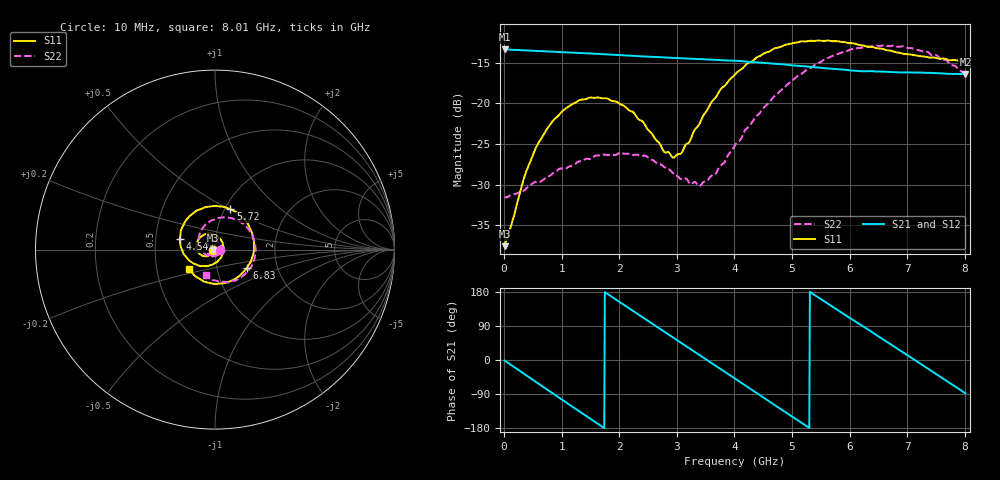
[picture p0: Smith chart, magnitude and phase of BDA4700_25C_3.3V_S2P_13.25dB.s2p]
!Agilent Technologies,E5071B,MY42404982,A.09.10
!Date: Mon Oct 20 18:08:35 2025
!Data & Calibration Information:
!Freq	S11:SOLT2(ON)	S21:SOLT2(ON)	S12:SOLT2(ON)	S22:SOLT2(ON)
# Hz S RI R 50
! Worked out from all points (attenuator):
!   801 points, 10 MHz to 8.01 GHz, reference 50 ohm
!   highest |S21| = -13.35 dB at 10 MHz (marker M1); lowest = -16.4 dB at 8.01 GHz (marker M2)
!   lowest |S11| = -37.6 dB at 10 MHz (marker M3), VSWR 1.03, Z = 48.7 - j0.149 ohm
!   |S11| at or under -10 dB: start of sweep to end of sweep
!   |S22| runs from -31.6 to -12.9 dB; largest |S21 - S12| = 0.0025
!   S11 on the Smith chart (normalised r, x): 10 MHz: 0.97, -0.00; 4.54 GHz: 0.67, +0.08; 5.72 GHz: 1.06, +0.51; 6.83 GHz: 1.40, -0.29; 8.01 GHz: 0.73, -0.16
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1e7  -0.0131 -0.00153  0.2149 -0.00476  0.2149 -0.00485  0.0265 -0.000952
3.6e8  -0.0242 -0.0264  0.167 -0.1299  0.1668 -0.1299  0.0221 -0.0193
5.8e8  -0.0419 -0.0366  0.1029 -0.1829  0.1028 -0.183  0.0135 -0.03
8.7e8  -0.072 -0.0334  -0.00215 -0.2076  -0.00199 -0.2076  -0.00897 -0.0365
1.35e9  -0.1043 0.0151  -0.1558 -0.1312  -0.1557 -0.1313  -0.0416 -0.0147
1.94e9  -0.0591 0.0839  -0.1863 0.0683  -0.1863 0.0683  -0.0328 0.0352
2.25e9  -0.0117 0.0868  -0.1215 0.1531  -0.1216 0.1533  -0.00804 0.0475
2.68e9  0.041 0.0405  0.0166 0.1915  0.0163 0.1914  0.0262 0.0334
2.96e9  0.0456 -0.00905  0.1036 0.1591  0.1035 0.1589  0.0348 0.0114
3.09e9  0.0386 -0.0318  0.137 0.1306  0.1357 0.1312  0.0341 -0.00103
3.4e9  -0.00172 -0.0754  0.1823 0.0409  0.1826 0.041  0.0187 -0.0249
3.67e9  -0.0568 -0.0921  0.1789 -0.0465  0.179 -0.047  -0.0061 -0.0363
4.01e9  -0.1342 -0.0676  0.1197 -0.1378  0.1199 -0.1375  -0.0459 -0.0304
4.54e9  -0.1963 0.0579  -0.0391 -0.1725  -0.0388 -0.1728  -0.09 0.0344
4.98e9  -0.1459 0.1813  -0.1438 -0.0932  -0.1442 -0.0939  -0.0713 0.1155
5.35e9  -0.0401 0.2386  -0.1667 0.0125  -0.1668 0.0115  -0.0064 0.1667
5.72e9  0.0853 0.2253  -0.1228 0.1069  -0.1226 0.107  0.0868 0.1765
6.23e9  0.2032 0.0995  0.00212 0.1573  0.00437 0.1574  0.1986 0.0951
6.68e9  0.2041 -0.0541  0.1109 0.1096  0.1113 0.1094  0.2232 -0.0283
6.83e9  0.1791 -0.1001  0.1344 0.0773  0.1348 0.0765  0.2121 -0.069
7.43e9  0.00691 -0.1908  0.1334 -0.0762  0.1333 -0.0766  0.0904 -0.1744
8.01e9  -0.1467 -0.1069  0.0051 -0.1511  0.00566 -0.1512  -0.0514 -0.141
